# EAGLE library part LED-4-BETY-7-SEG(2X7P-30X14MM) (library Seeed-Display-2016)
304080005
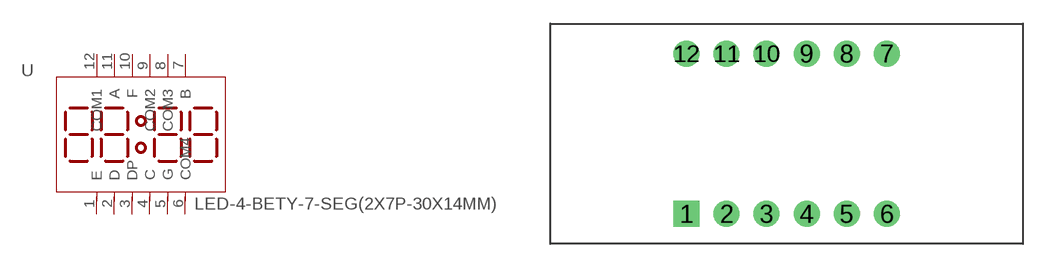
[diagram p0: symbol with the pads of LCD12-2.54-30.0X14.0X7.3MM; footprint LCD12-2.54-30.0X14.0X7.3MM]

Designator prefix U

## LED-4-BETY-7-SEG(2X7P-30X14MM) (MPN: SYD3642ASR; VALUE: SYD3642ASR)  [LCD12-2.54-30.0X14.0X7.3MM]
1  E
2  D
3  DP
4  C
5  G
6  COM4
7  B
8  COM3
9  COM2
10  F
11  A
12  COM1

## Footprint LCD12-2.54-30.0X14.0X7.3MM (pad centres in mm)
drill 0.889 pad 1.651 square: 1 -6.35,-5.08
drill 0.889 pad 1.651: 2 -3.81,-5.08; 3 -1.27,-5.08; 4 1.27,-5.08; 5 3.81,-5.08; 6 6.35,-5.08; 7 6.35,5.08; 8 3.81,5.08; 9 1.27,5.08; 10 -1.27,5.08; 11 -3.81,5.08; 12 -6.35,5.08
